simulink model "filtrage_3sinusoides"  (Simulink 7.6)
settings: Solver=ode15s  StartTime=0.0  StopTime=0.005  RelTol=1e-3
InitFcn:
  | clc, clear all
StopFcn:
  | delete *.mat
  | delete *.asv
libraries: fl_lib x21, nesl_utility x4

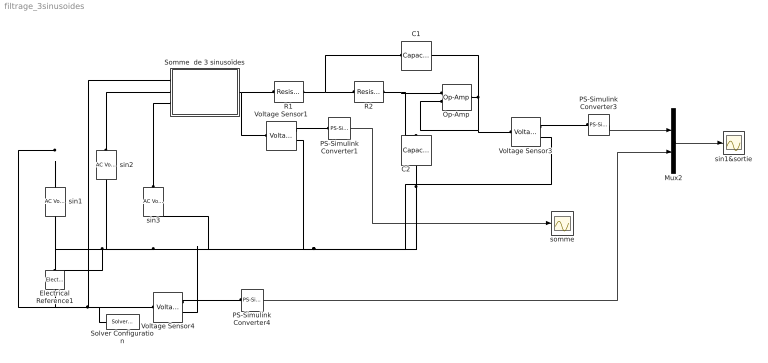
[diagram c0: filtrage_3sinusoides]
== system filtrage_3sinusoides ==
  C1 : fl_lib/Electrical/Electrical Elements/Capacitor  DialogController=NetworkEngine.DynNeDlgSource  SystemSampleTime=-1  c=0.04 uF  v0=1 V  r=1e-6 Ohm  g=0 1/Ohm  i_Log=off  v_Log=off  vc_Log=off  LocalVarNames=|i|v|vc  LocalVarDescs=|i|v|Internal variable for voltage across capacitor term  LocalVarLogging=[0 0 0]
  C2 : fl_lib/Electrical/Electrical Elements/Capacitor  DialogController=NetworkEngine.DynNeDlgSource  SystemSampleTime=-1  c=0.04 uF  v0=1 V  r=1e-6 Ohm  g=0 1/Ohm  i_Log=off  v_Log=off  vc_Log=off  LocalVarNames=|i|v|vc  LocalVarDescs=|i|v|Internal variable for voltage across capacitor term  LocalVarLogging=[0 0 0]
  Electrical Reference1 : fl_lib/Electrical/Electrical Elements/Electrical Reference  DialogController=NetworkEngine.DynNeDlgSource  SystemSampleTime=-1  i_Log=off  LocalVarNames=|i  LocalVarDescs=|i  LocalVarLogging=[]
  Mux2 : Mux  Inputs=2
  Op-Amp : fl_lib/Electrical/Electrical Elements/Op-Amp  DialogController=NetworkEngine.DynNeDlgSource  SystemSampleTime=-1  i1_Log=off  v1_Log=off  outI_Log=off  LocalVarNames=|i1|v1|outI  LocalVarDescs=|i1|v1|outI  LocalVarLogging=[]
  PS-Simulink Converter1 : nesl_utility/PS-Simulink Converter  DialogController=NetworkEngine.DynNeUtilDlgSource  SystemSampleTime=-1  PhysicalDomain=network_engine_domain  LeftPortType=input  RightPortType=output  SubClassName=ps_output  Unit=1  AffineConversion=off
  PS-Simulink Converter3 : nesl_utility/PS-Simulink Converter  DialogController=NetworkEngine.DynNeUtilDlgSource  SystemSampleTime=-1  PhysicalDomain=network_engine_domain  LeftPortType=input  RightPortType=output  SubClassName=ps_output  Unit=1  AffineConversion=off
  PS-Simulink Converter4 : nesl_utility/PS-Simulink Converter  DialogController=NetworkEngine.DynNeUtilDlgSource  SystemSampleTime=-1  PhysicalDomain=network_engine_domain  LeftPortType=input  RightPortType=output  SubClassName=ps_output  Unit=1  AffineConversion=off
  R1 : fl_lib/Electrical/Electrical Elements/Resistor  DialogController=NetworkEngine.DynNeDlgSource  SystemSampleTime=-1  R=1 kOhm  i_Log=off  v_Log=off  LocalVarNames=|current|voltage|power  LocalVarDescs=|Resistor current (A)|Voltage across resistor (V)|Power (W)  LocalVarLogging=[0 0 0]
  R2 : fl_lib/Electrical/Electrical Elements/Resistor  DialogController=NetworkEngine.DynNeDlgSource  SystemSampleTime=-1  R=1 kOhm  i_Log=off  v_Log=off  LocalVarNames=|current|voltage|power  LocalVarDescs=|Resistor current (A)|Voltage across resistor (V)|Power (W)  LocalVarLogging=[0 0 0]
  Solver Configuration : nesl_utility/Solver Configuration  DialogController=NetworkEngine.DynNeUtilDlgSource  SystemSampleTime=-1  PhysicalDomain=network_engine_domain  LeftPortType=input  RightPortType=generic  SubClassName=solver  Accelerate=off  Profile=off  ResidualTolerance=1e-9  MaxNonlinIter=12  MaxModeIter=2  DoFixedCost=off  UseLocalSampling=off  DoDC=off  LinearAlgebra=Sparse  LocalSolverSampleTime=.001  LocalSolverChoice=NE_BACKWARD_EULER_ADVANCER  UseLocalSolver=off
  Somme  de 3 sinusoïdes : Subsystem
  Voltage Sensor1 : fl_lib/Electrical/Electrical Sensors/Voltage Sensor  DialogController=NetworkEngine.DynNeDlgSource  SystemSampleTime=-1  i1_Log=off  v1_Log=off  LocalVarNames=|i1|v1  LocalVarDescs=|i1|v1  LocalVarLogging=[]
  Voltage Sensor3 : fl_lib/Electrical/Electrical Sensors/Voltage Sensor  DialogController=NetworkEngine.DynNeDlgSource  SystemSampleTime=-1  i1_Log=off  v1_Log=off  LocalVarNames=|i1|v1  LocalVarDescs=|i1|v1  LocalVarLogging=[]
  Voltage Sensor4 : fl_lib/Electrical/Electrical Sensors/Voltage Sensor  DialogController=NetworkEngine.DynNeDlgSource  SystemSampleTime=-1  i1_Log=off  v1_Log=off  LocalVarNames=|i1|v1  LocalVarDescs=|i1|v1  LocalVarLogging=[]
  sin1 : fl_lib/Electrical/Electrical Sources/AC Voltage Source  DialogController=NetworkEngine.DynNeDlgSource  SystemSampleTime=-1  amp=1 V  shift=pi/2 rad  omega=1 kHz  i_Log=off  v_Log=off  LocalVarNames=|i|v  LocalVarDescs=|i|v  LocalVarLogging=[0 0]
  sin1&sortie : Scope
  sin2 : fl_lib/Electrical/Electrical Sources/AC Voltage Source  DialogController=NetworkEngine.DynNeDlgSource  SystemSampleTime=-1  amp=5 V  shift=2*pi/3 rad  omega=100 kHz  i_Log=off  v_Log=off  LocalVarNames=|i|v  LocalVarDescs=|i|v  LocalVarLogging=[0 0]
  sin3 : fl_lib/Electrical/Electrical Sources/AC Voltage Source  DialogController=NetworkEngine.DynNeDlgSource  SystemSampleTime=-1  amp=10 V  shift=2*pi/5 rad  omega=125 kHz  i_Log=off  v_Log=off  LocalVarNames=|i|v  LocalVarDescs=|i|v  LocalVarLogging=[0 0]
  somme : Scope
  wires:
  PS-Simulink Converter3/1 -> Mux2/1
  PS-Simulink Converter1/1 -> somme/1
  Mux2/1 -> sin1&sortie/1
  PS-Simulink Converter4/1 -> Mux2/2
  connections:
  C2/RConn1 -- Voltage Sensor3/RConn2 -- Voltage Sensor1/RConn2 -- sin2/RConn1 -- sin1/RConn1 -- Electrical Reference1/LConn1 -- sin3/RConn1 -- Voltage Sensor4/RConn2
  R2/RConn1 -- C2/LConn1 -- Op-Amp/LConn1
  R1/RConn1 -- R2/LConn1 -- C1/LConn1
  Op-Amp/RConn1 -- C1/RConn1 -- Voltage Sensor3/LConn1 -- Op-Amp/LConn2
  Voltage Sensor3/RConn1 -- PS-Simulink Converter3/LConn1
  sin3/LConn1 -- Somme  de 3 sinusoïdes/LConn3
  sin2/LConn1 -- Somme  de 3 sinusoïdes/LConn2
  sin1/LConn1 -- Somme  de 3 sinusoïdes/LConn1 -- Voltage Sensor4/LConn1 -- Solver Configuration/RConn1
  Somme  de 3 sinusoïdes/RConn1 -- R1/LConn1 -- Voltage Sensor1/LConn1
  Voltage Sensor1/RConn1 -- PS-Simulink Converter1/LConn1
  Voltage Sensor4/RConn1 -- PS-Simulink Converter4/LConn1

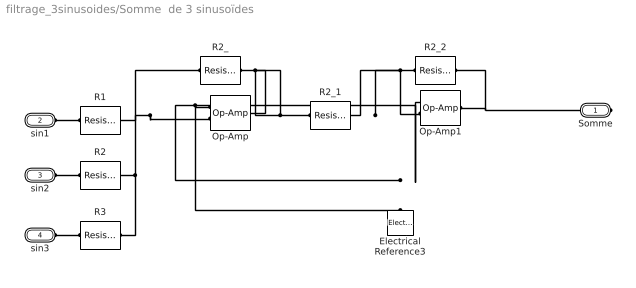
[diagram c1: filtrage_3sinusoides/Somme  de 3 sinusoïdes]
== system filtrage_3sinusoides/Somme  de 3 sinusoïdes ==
  Electrical Reference3 : fl_lib/Electrical/Electrical Elements/Electrical Reference  DialogController=NetworkEngine.DynNeDlgSource  SystemSampleTime=-1  i_Log=off  LocalVarNames=|i  LocalVarDescs=|i  LocalVarLogging=[]
  Op-Amp : fl_lib/Electrical/Electrical Elements/Op-Amp  DialogController=NetworkEngine.DynNeDlgSource  SystemSampleTime=-1  i1_Log=off  v1_Log=off  outI_Log=off  LocalVarNames=|i1|v1|outI  LocalVarDescs=|i1|v1|outI  LocalVarLogging=[]
  Op-Amp1 : fl_lib/Electrical/Electrical Elements/Op-Amp  DialogController=NetworkEngine.DynNeDlgSource  SystemSampleTime=-1  i1_Log=off  v1_Log=off  outI_Log=off  LocalVarNames=|i1|v1|outI  LocalVarDescs=|i1|v1|outI  LocalVarLogging=[]
  R1 : fl_lib/Electrical/Electrical Elements/Resistor  DialogController=NetworkEngine.DynNeDlgSource  SystemSampleTime=-1  R=10 kOhm  i_Log=off  v_Log=off  LocalVarNames=|current|voltage|power  LocalVarDescs=|Resistor current (A)|Voltage across resistor (V)|Power (W)  LocalVarLogging=[0 0 0]
  R2 : fl_lib/Electrical/Electrical Elements/Resistor  DialogController=NetworkEngine.DynNeDlgSource  SystemSampleTime=-1  R=10 kOhm  i_Log=off  v_Log=off  LocalVarNames=|current|voltage|power  LocalVarDescs=|Resistor current (A)|Voltage across resistor (V)|Power (W)  LocalVarLogging=[0 0 0]
  R2_ : fl_lib/Electrical/Electrical Elements/Resistor  DialogController=NetworkEngine.DynNeDlgSource  SystemSampleTime=-1  R=10 kOhm  i_Log=off  v_Log=off  LocalVarNames=|current|voltage|power  LocalVarDescs=|Resistor current (A)|Voltage across resistor (V)|Power (W)  LocalVarLogging=[0 0 0]
  R2_1 : fl_lib/Electrical/Electrical Elements/Resistor  DialogController=NetworkEngine.DynNeDlgSource  SystemSampleTime=-1  R=10 kOhm  i_Log=off  v_Log=off  LocalVarNames=|current|voltage|power  LocalVarDescs=|Resistor current (A)|Voltage across resistor (V)|Power (W)  LocalVarLogging=[0 0 0]
  R2_2 : fl_lib/Electrical/Electrical Elements/Resistor  DialogController=NetworkEngine.DynNeDlgSource  SystemSampleTime=-1  R=10 kOhm  i_Log=off  v_Log=off  LocalVarNames=|current|voltage|power  LocalVarDescs=|Resistor current (A)|Voltage across resistor (V)|Power (W)  LocalVarLogging=[0 0 0]
  R3 : fl_lib/Electrical/Electrical Elements/Resistor  DialogController=NetworkEngine.DynNeDlgSource  SystemSampleTime=-1  R=10 kOhm  i_Log=off  v_Log=off  LocalVarNames=|current|voltage|power  LocalVarDescs=|Resistor current (A)|Voltage across resistor (V)|Power (W)  LocalVarLogging=[0 0 0]
  Somme : PMIOPort  Port=1  Side=Right
  sin1 : PMIOPort  Port=2  Side=Left
  sin2 : PMIOPort  Port=3  Side=Left
  sin3 : PMIOPort  Port=4  Side=Left
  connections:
  sin3/RConn1 -- R3/LConn1
  sin2/RConn1 -- R2/LConn1
  sin1/RConn1 -- R1/LConn1
  R2_2/RConn1 -- Somme/RConn1 -- Op-Amp1/RConn1
  R2_2/LConn1 -- Op-Amp1/LConn2 -- R2_1/RConn1
  R2_/RConn1 -- R2_1/LConn1 -- Op-Amp/RConn1
  R3/RConn1 -- R2_/LConn1 -- Op-Amp/LConn2 -- R1/RConn1 -- R2/RConn1
  Op-Amp/LConn1 -- Electrical Reference3/LConn1 -- Op-Amp1/LConn1
